(* Logix 5000 Controller export DL232_Example; controller DL232_Example 1756-L75 rev 19.13; software revision 19.01 *)

TASK MainTask (continuous, watchdog 500 ms) : MainProgram

MODULES
   Local : 1756-L75 (ICP 0, rev 19.13)
      EtherNet_Bridge : 1756-EN2TR (ICP 1, Ethernet 192.168.1.6, rev 3.6)
         DL232 : ETHERNET-MODULE (Ethernet 192.168.1.173, rev 1.1, Output RPI 500 ms)
END_MODULES

TYPE ProSoftPLX51DL232DataSource :
STRUCT
   EtherNetIP : BOOL;
   DF1 : BOOL;
   ModbusRTU : BOOL;
   ModbusTCP : BOOL;
END_STRUCT
END_TYPE

TYPE ProSoftPLX51DL232Input :
STRUCT
   Instance : STRING;
   Status : ProSoftPLX51DL232Status;
   CachePercentageUsed : REAL;
   CacheRecordCount : DINT;
   TotalRecordCount : DINT;
   ActiveTagCount : DINT;
   DataSource : ProSoftPLX51DL232DataSource;
   DataSourceReadCount : DINT;
END_STRUCT
END_TYPE

TYPE ProSoftPLX51DL232Status :
STRUCT
   Running : BOOL;
   ConfigurationValid : BOOL;
   ContinuousLogging : BOOL;
   LogRollover : BOOL;
   LoggingInhibited : BOOL;
   LoggingStopped : BOOL;
END_STRUCT
END_TYPE

VAR_GLOBAL   (* controller tags *)
   DL232Input : ProSoftPLX51DL232Input := (Instance := 'Data Logger', Status.Running := 1, Status.ConfigurationValid := 1, Status.ContinuousLogging := 1, CachePercentageUsed := 5.96046448e-004, CacheRecordCount := 100, TotalRecordCount := 100, ActiveTagCount := 100, DataSource.EtherNetIP := 1, DataSourceReadCount := 4000);
END_VAR

PROGRAM MainProgram   (* main routine MainRoutine *)

ROUTINE DL232_Routine   (* ladder *)
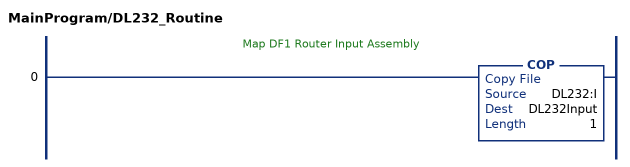
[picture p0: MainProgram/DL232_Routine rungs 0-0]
   // Map DF1 Router Input Assembly
   0: COP(DL232:I,DL232Input,1);
END_ROUTINE

ROUTINE MainRoutine   (* ladder *)
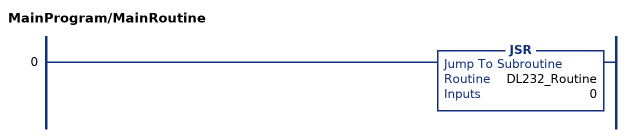
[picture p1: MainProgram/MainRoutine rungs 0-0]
   0: JSR(DL232_Routine,0);
END_ROUTINE
END_PROGRAM
